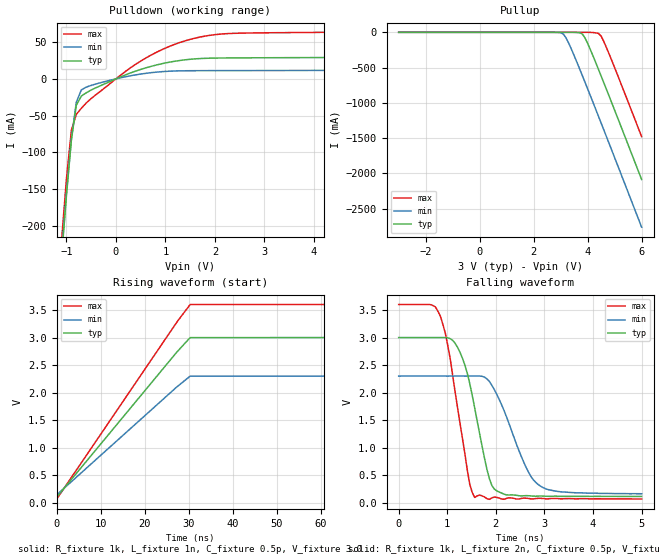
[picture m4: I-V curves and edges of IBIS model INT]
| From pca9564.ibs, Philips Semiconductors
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[Model]   INT
Model_type Output
C_comp   0.5p   0.5p   0.5p
[Temperature Range] 27   85   -40
[Voltage Range]   3   2.3   3.6
[Pullup Reference]  3   2.3   3.6
[Pulldown Reference]0   0   0
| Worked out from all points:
|   slope of the pulldown table from 0 to 0.45 V, typ, clamps not added: 38.4 ohm
|   falling waveform, R_fixture 1k, L_fixture 2n, C_fixture 0.5p, V_fixture 3.0: 20-80 % time 408ps typ, 581ps min, 380ps max; typ from 3 V to 0.112 V
|   rising waveform, R_fixture 1k, L_fixture 1n, C_fixture 0.5p, V_fixture 3.0: 20-80 % time 18ns typ, 18ns min, 18ns max; typ from 0.097 V to 3 V
[Pullup]
-3V       73.89pA    109.4pA    67.15pA
2.7V      1.665pA    -56.9uA    3.897pA
3V        -11.87pA   -5.075mA   234.7fA
3.1V      -485.9pA   -24.76mA   -985.4fA
3.3V      -1.044uA   -154.5mA   -3.424pA
3.7V      -5.255mA   -514.5mA   -59.79pA
3.8V      -22.13mA   -609.1mA   -4.837nA
4V        -156.3mA   -800.4mA   -24.46uA
4.4V      -522.6mA   -1.188A    -14.84mA
4.5V      -618.1mA   -1.285A    -53.46mA
4.9V      -1.005A    -1.677A    -404.9mA
6V        -2.086A    -2.761A    -1.478A
[Pulldown]
-3V       -2.086A    -2.071A    -2.071A
-1.1V     -245.6mA   -240.8mA   -222.1mA
-1V       -159.4mA   -156.3mA   -136.8mA
-900mV    -83.43mA   -81.92mA   -70.2mA
-800mV    -35.9mA    -31.78mA   -48.38mA
-700mV    -23.54mA   -15.1mA    -40.21mA
-600mV    -19.04mA   -11.2mA    -32.89mA
600mV     14.93mA    7.523mA    28.27mA
1.1V      23mA       10.53mA    44.8mA
1.6V      27.28mA    11.16mA    55.55mA
2.3V      28.57mA    11.29mA    61.89mA
6V        32.34mA    13.42mA    68.48mA
[Falling Waveform]
R_fixture=1k
L_fixture=2n
C_fixture=0.5p
V_fixture=3.0
V_fixture_min=2.3
V_fixture_max=3.6
0s        3V         2.3V       3.6V
858.6ps   3V         2.3V       3.387V
1.061ns   2.979V     2.3V       2.617V
1.263ns   2.73V      2.3V       1.441V
1.465ns   2.157V     2.3V       326.3mV
1.566ns   1.716V     2.3V       93.9mV
1.818ns   599mV      2.247V     70.92mV
2.02ns    214.3mV    1.964V     95.48mV
2.879ns   119.8mV    325.1mV    78.63mV
5ns       112.4mV    161.9mV    67.17mV
[Rising Waveform]
R_fixture=1k
L_fixture=1n
C_fixture=0.5p
V_fixture=3.0
V_fixture_min=2.3
V_fixture_max=3.6
0s        97.22mV    139.3mV    61.41mV
27.27ns   2.735V     2.102V     3.278V
30.3ns    2.998V     2.299V     3.599V
300ns     3V         2.3V       3.6V
[Ramp]
R_load=1k
dV/dt_r   1.733E+0/3.043E-10   1.283E+0/6.513E-10   2.120E+0/1.782E-10
dV/dt_f   1.733E+0/4.040E-10   1.283E+0/5.012E-10   2.120E+0/4.213E-10
|[End   INT
